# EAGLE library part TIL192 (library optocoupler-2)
TEXAS INSTRUMENTS OPTO COUPLER
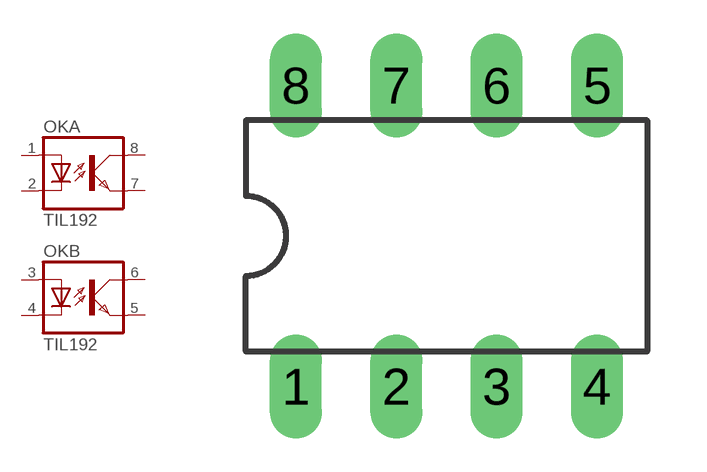
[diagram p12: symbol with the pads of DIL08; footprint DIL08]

Designator prefix OK; gates A=OK B=OK

## TIL192  [DIL08]
1  A:A  pas
2  A:C  pas
3  B:A  pas
4  B:C  pas
5  B:EMIT  pas
6  B:COL  pas
7  A:EMIT  pas
8  A:COL  pas

## Footprint DIL08 (pad centres in mm)
Dual In Line Package
drill 0.813 long: 1 -3.81,-3.81; 2 -1.27,-3.81; 3 1.27,-3.81; 4 3.81,-3.81; 5 3.81,3.81; 6 1.27,3.81; 7 -1.27,3.81; 8 -3.81,3.81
